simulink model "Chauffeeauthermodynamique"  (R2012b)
settings: Solver=ode45  StartTime=0.0  StopTime=60000  RelTol=1e-3
libraries: fl_lib x9, nesl_utility x6

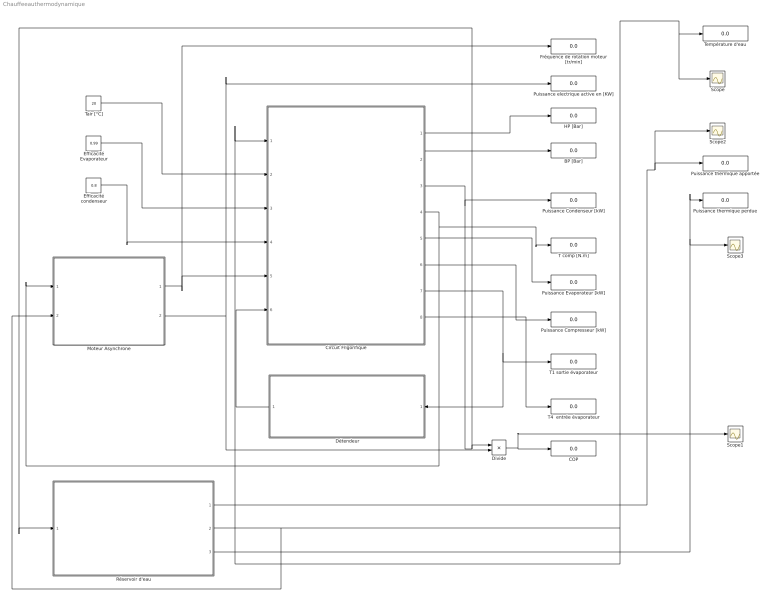
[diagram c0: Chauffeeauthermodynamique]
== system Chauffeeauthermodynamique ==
  BP [Bar] : Display
  COP : Display
  Circuit Frigorifique : Subsystem
  Divide : Product  Inputs=*/
  Détendeur : Subsystem
  Efficacité Evaporateur : Constant  Value=0.99
  Efficacité condenseur : Constant  Value=0.8
  Fréquence de rotation moteur [tr/min] : Display
  HP [Bar] : Display
  Moteur Asynchrone : Subsystem
  Puissance Compresseur [kW] : Display
  Puissance Condenseur [kW] : Display
  Puissance Evaporateur [kW] : Display
  Puissance electrique active en [KW] : Display
  Puissance thermique apportée : Display
  Puissance thermique perdue : Display
  Réservoir d'eau : Subsystem
  Scope{,1..3} (4 alike) : Scope
  T comp [N.m] : Display
  T1 sortie évaporateur : Display
  T4  entrée évaporateur : Display
  Tair [°C] : Constant  Value=20
  Température d'eau : Display
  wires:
  Efficacité Evaporateur/1 -> Circuit Frigorifique/3(Eff Evapo)
  Circuit Frigorifique/1(HP [bar]) -> HP [Bar]/1
  Circuit Frigorifique/2(BP [bar]) -> BP [Bar]/1
  Circuit Frigorifique/4(Tm [N.m]) -> Moteur Asynchrone/1(Tm [N.m]), T comp [N.m]/1
  Circuit Frigorifique/8(T4 [°C]) -> T4  entrée évaporateur/1
  Circuit Frigorifique/7(T1 [°C]) -> Détendeur/1(T1), T1 sortie évaporateur/1
  Circuit Frigorifique/5(Pevapo [kW]) -> Puissance Evaporateur [kW]/1
  Divide/1 -> Scope1/1, COP/1
  Circuit Frigorifique/6(Pcomp [kW]) -> Puissance Compresseur [kW]/1
  Efficacité condenseur/1 -> Circuit Frigorifique/4(effc)
  Détendeur/1(BP [Bar]) -> Circuit Frigorifique/6(BP[Bar])
  Moteur Asynchrone/2(Puissance Electrique active [W]) -> Puissance electrique active en [KW]/1, Divide/2
  Moteur Asynchrone/1(N [tr/min]) -> Fréquence de rotation moteur [tr/min]/1, Circuit Frigorifique/5(N [tr/min])
  Tair [°C]/1 -> Circuit Frigorifique/2(Tair [°C])
  Circuit Frigorifique/3(Pcond [kW]) -> Réservoir d'eau/1(" Puissance Condenseur [kW]"), Divide/1, Puissance Condenseur [kW]/1
  Réservoir d'eau/2(Température du réservoir [°C]) -> Moteur Asynchrone/2(Teau [°C]), Scope/1, Température d'eau/1, Circuit Frigorifique/1(Tee [°C])
  Réservoir d'eau/1(Puissance Condenseur [W]) -> Scope2/1, Puissance thermique apportée/1
  Réservoir d'eau/3(Puissance thermique perdue [W]) -> Scope3/1, Puissance thermique perdue/1

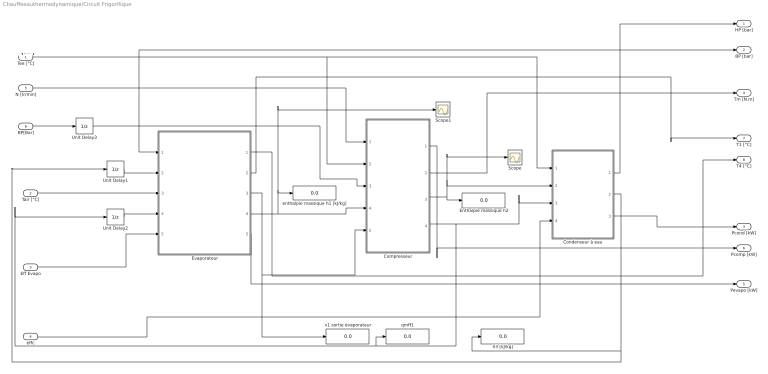
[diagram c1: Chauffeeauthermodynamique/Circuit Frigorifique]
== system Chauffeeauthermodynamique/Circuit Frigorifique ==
  note: +++++
  Tee [°C] : Inport
  Tair [°C] : Inport  Port=2
  Eff Evapo : Inport  Port=3
  effc : Inport  Port=4
  N [tr/min] : Inport  Port=5
  BP[Bar] : Inport  Port=6
  Compresseur : Subsystem
  Condenseur à eau : Subsystem
  Enthalpie massique h2 : Display
  Evaporateur : Subsystem
  Scope : Scope
  Scope1 : Scope
  Unit Delay1 : UnitDelay  InitialCondition=300  SampleTime=-1
  Unit Delay2 : UnitDelay  InitialCondition=0.00001  SampleTime=-1
  Unit Delay3 : UnitDelay  InitialCondition=2.5  SampleTime=-1
  enthalpie massique h1 [kJ/kg] : Display
  h3 [kJ/kg] : Display
  qmff1 : Display
  v1 sortie évaporateur : Display
  HP [bar] : Outport
  BP [bar] : Outport  Port=2
  Pcond [kW] : Outport  Port=3
  Tm [N.m] : Outport  Port=4
  Pevapo [kW] : Outport  Port=5
  Pcomp [kW] : Outport  Port=6
  T1 [°C] : Outport  Port=7
  T4 [°C] : Outport  Port=8
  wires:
  Evaporateur/2(T1 [°C]) -> T1 [°C]/1
  N [tr/min]/1 -> Compresseur/1(N [tr/min])
  Evaporateur/5(Pévapo [kW]) -> Pevapo [kW]/1
  Tair [°C]/1 -> Evaporateur/3(Tair [°C])
  Unit Delay2/1 -> Evaporateur/4(qmff [kg/s])
  Condenseur à eau/1(HP [bar]) -> HP [bar]/1
  BP[Bar]/1 -> Unit Delay3/1
  Compresseur/4(qmff [kg/s]) -> Unit Delay2/1, qmff1/1, Condenseur à eau/3(qmff [kg/s])
  Tee [°C]/1 -> Compresseur/2(Tee [°C]), Condenseur à eau/1(Tee [°C])
  Eff Evapo/1 -> Evaporateur/5(Eff)
  Evaporateur/3(v1 [m3/kg]) -> v1 sortie évaporateur/1, Compresseur/5(v1 [m3/kg])
  Condenseur à eau/2(h3 [kJ/kg]) -> Unit Delay1/1, h3 [kJ/kg]/1
  Evaporateur/4(h1 [kJ/kg]) -> Compresseur/4(h1 [kJ/kg]), Scope1/1, enthalpie massique h1 [kJ/kg]/1
  Compresseur/3(h2 [kJ/kg]) -> Scope/1, Condenseur à eau/2(h2 [kJ/kg]), Enthalpie massique h2/1
  Compresseur/2(Tm [N.m]) -> Tm [N.m]/1
  Evaporateur/1(T4 [°C]) -> T4 [°C]/1
  Condenseur à eau/3(Pcond [kW]) -> Pcond [kW]/1
  Unit Delay1/1 -> Evaporateur/2(h3 [kJ/kg])
  Compresseur/1(Pcomp [kW]) -> Pcomp [kW]/1
  effc/1 -> Condenseur à eau/4(effc)
  Unit Delay3/1 -> BP [bar]/1, Compresseur/3(BP [bar]), Evaporateur/1(BP [bar])

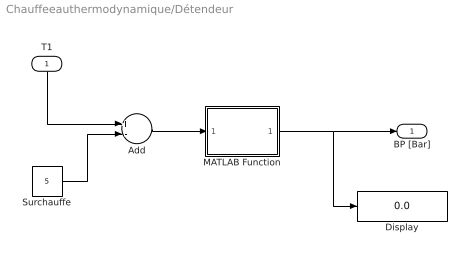
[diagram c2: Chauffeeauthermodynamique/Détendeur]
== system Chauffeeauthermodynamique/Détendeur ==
  T1 : Inport
  Add : Sum  Inputs=+-
  Display : Display
  MATLAB Function : MATLAB Function  TreatAsAtomicUnit=on
  Surchauffe : Constant  Value=5
  BP [Bar] : Outport
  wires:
  Add/1 -> MATLAB Function/1(T)
  T1/1 -> Add/1
  Surchauffe/1 -> Add/2
  MATLAB Function/1(BP) -> Display/1, BP [Bar]/1

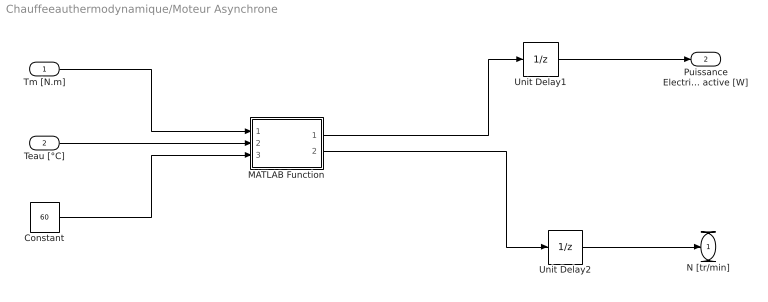
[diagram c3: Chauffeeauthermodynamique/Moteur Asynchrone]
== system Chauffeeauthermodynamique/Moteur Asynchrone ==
  Tm [N.m] : Inport
  Teau [°C] : Inport  Port=2
  Constant : Constant  Value=60
  MATLAB Function : MATLAB Function  TreatAsAtomicUnit=on
  Unit Delay1 : UnitDelay  InitialCondition=0.2  SampleTime=-1
  Unit Delay2 : UnitDelay  SampleTime=-1
  N [tr/min] : Outport
  Puissance Electrique active [W] : Outport  Port=2
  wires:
  Tm [N.m]/1 -> MATLAB Function/1(Tm)
  MATLAB Function/1(P) -> Unit Delay1/1
  MATLAB Function/2(N) -> Unit Delay2/1
  Unit Delay1/1 -> Puissance Electrique active [W]/1
  Unit Delay2/1 -> N [tr/min]/1
  Teau [°C]/1 -> MATLAB Function/2(Teau)
  Constant/1 -> MATLAB Function/3(Tcons)

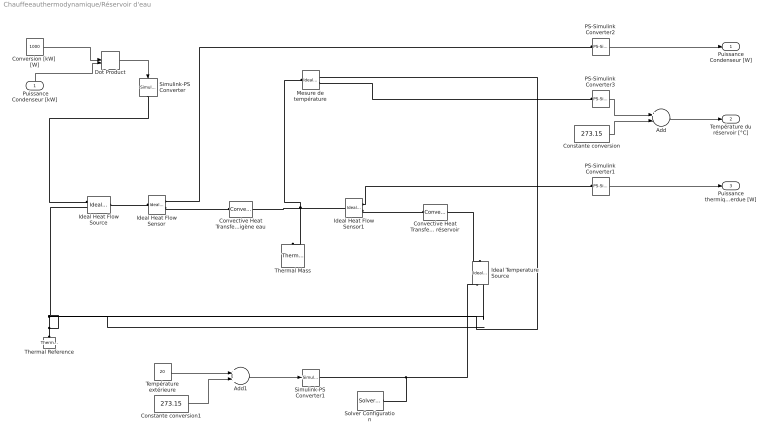
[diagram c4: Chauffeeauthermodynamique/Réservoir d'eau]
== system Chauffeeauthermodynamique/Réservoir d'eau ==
  " Puissance Condenseur [kW]" : Inport
  Add : Sum  Inputs=+-
  Add1 : Sum
  Constante conversion : Constant  Value=273.15
  Constante conversion1 : Constant  Value=273.15
  Convective Heat Transfer Echange Fluide frigorigène eau : fl_lib/Thermal/Thermal Elements/Convective Heat Transfer  area=0.82 m^2  heat_tr_coeff=25 W/(m^2 * K)  Q_Log=off  T_Log=off  LocalVarNames=|Q|T  LocalVarDescs=|Q|T  LocalVarLogging=[0 0]
  Convective Heat Transfer1 Echange avec l'extérieur du réservoir : fl_lib/Thermal/Thermal Elements/Convective Heat Transfer  area=1 m^2  heat_tr_coeff=0.0015 W/(m^2 * K)  Q_Log=off  T_Log=off  LocalVarNames=|Q|T  LocalVarDescs=|Q|T  LocalVarLogging=[0 0]
  Conversion [kW]  [W] : Constant  Value=1000
  Dot Product : DotProduct
  Ideal Heat Flow Sensor : fl_lib/Thermal/Thermal Sensors/Ideal Heat Flow Sensor  Q_Log=off  T_Log=off  LocalVarNames=|Q|T  LocalVarDescs=|Q|T  LocalVarLogging=[0 0]
  Ideal Heat Flow Sensor1 : fl_lib/Thermal/Thermal Sensors/Ideal Heat Flow Sensor  Q_Log=off  T_Log=off  LocalVarNames=|Q|T  LocalVarDescs=|Q|T  LocalVarLogging=[0 0]
  Ideal Heat Flow Source : fl_lib/Thermal/Thermal Sources/Ideal Heat Flow Source  Q_Log=off  T_Log=off  LocalVarNames=|Q|T  LocalVarDescs=|Q|T  LocalVarLogging=[0 0]
  Ideal Temperature Source : fl_lib/Thermal/Thermal Sources/Ideal Temperature Source  Q_Log=off  T_Log=off  LocalVarNames=|Q|T  LocalVarDescs=|Q|T  LocalVarLogging=[0 0]
  Mesure de température : fl_lib/Thermal/Thermal Sensors/Ideal Temperature Sensor  Qs_Log=off  Ts_Log=off  LocalVarNames=|Qs|Ts  LocalVarDescs=|Qs|Ts  LocalVarLogging=[]
  PS-Simulink Converter1 : nesl_utility/PS-Simulink Converter  PhysicalDomain=network_engine_domain  LeftPortType=input  RightPortType=output  SubClassName=ps_output  PseudoPeriodic=off  Frequencies=[]  Unit=1  AffineConversion=off
  PS-Simulink Converter2 : nesl_utility/PS-Simulink Converter  PhysicalDomain=network_engine_domain  LeftPortType=input  RightPortType=output  SubClassName=ps_output  PseudoPeriodic=off  Frequencies=[]  Unit=1  AffineConversion=off
  PS-Simulink Converter3 : nesl_utility/PS-Simulink Converter  PhysicalDomain=network_engine_domain  LeftPortType=input  RightPortType=output  SubClassName=ps_output  PseudoPeriodic=off  Frequencies=[]  Unit=1  AffineConversion=off
  Simulink-PS Converter : nesl_utility/Simulink-PS Converter  PhysicalDomain=network_engine_domain  LeftPortType=input  RightPortType=output  SubClassName=ps_input  PseudoPeriodic=off  Frequencies=[]  NoiseDistribution=none  NoiseParameters=[]  Unit=1  AffineConversion=off  InputFilterTimeConstant=.001  UdotUserProvided=1  SimscapeFilterOrder=1  InputFiltering=off
  Simulink-PS Converter1 : nesl_utility/Simulink-PS Converter  PhysicalDomain=network_engine_domain  LeftPortType=input  RightPortType=output  SubClassName=ps_input  PseudoPeriodic=off  Frequencies=[]  NoiseDistribution=none  NoiseParameters=[]  Unit=K  AffineConversion=on  InputFilterTimeConstant=.001  UdotUserProvided=1  SimscapeFilterOrder=1  InputFiltering=off
  Solver Configuration : nesl_utility/Solver Configuration  PhysicalDomain=network_engine_domain  LeftPortType=input  RightPortType=generic  SubClassName=solver  Accelerate=off  Profile=off  UseLocalSampling=off  FrequencyDomain=off  Tones=[]  Harmonics=[]  UseCCode=off  SimulateNoise=off  EnableSwitchedLinearOptims=on  DoDC=off  ResidualTolerance=1e-9  UseLocalSolver=off  LocalSolverChoice=NE_BACKWARD_EULER_ADVANCER  LocalSolverSampleTime=.001  DoFixedCost=off  MaxNonlinIter=3  MaxModeIter=2  LinearAlgebra=Sparse  DelaysMemoryBudget=1024
  Température extérieure : Constant  Value=20
  Thermal Mass : fl_lib/Thermal/Thermal Elements/Thermal Mass  mass=200 kg  sp_heat=4185 J/kg/K  init_temp=15 C  Q_Log=off  LocalVarNames=|Q  LocalVarDescs=|Q  LocalVarLogging=0
  Thermal Reference : fl_lib/Thermal/Thermal Elements/Thermal Reference  Q_Log=off  LocalVarNames=|Q  LocalVarDescs=|Q  LocalVarLogging=0
  Puissance Condenseur [W] : Outport
  Température du réservoir [°C] : Outport  Port=2
  Puissance thermique perdue [W] : Outport  Port=3
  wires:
  " Puissance Condenseur [kW]"/1 -> Dot Product/2
  PS-Simulink Converter3/1 -> Add/1
  Add/1 -> Température du réservoir [°C]/1
  Constante conversion/1 -> Add/2
  Dot Product/1 -> Simulink-PS Converter/1
  Conversion [kW]  [W]/1 -> Dot Product/1
  PS-Simulink Converter1/1 -> Puissance thermique perdue [W]/1
  PS-Simulink Converter2/1 -> Puissance Condenseur [W]/1
  Add1/1 -> Simulink-PS Converter1/1
  Température extérieure/1 -> Add1/1
  Constante conversion1/1 -> Add1/2
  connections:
  Thermal Reference/LConn1 -- Ideal Temperature Source/RConn2 -- Mesure de température/RConn1 -- Ideal Heat Flow Source/RConn2
  Mesure de température/LConn1 -- Thermal Mass/LConn1 -- Ideal Heat Flow Sensor1/LConn1 -- Convective Heat Transfer Echange Fluide frigorigène eau/RConn1
  Solver Configuration/RConn1 -- Ideal Temperature Source/RConn1 -- Simulink-PS Converter1/RConn1
  Simulink-PS Converter/RConn1 -- Ideal Heat Flow Source/RConn1
  Convective Heat Transfer1 Echange avec l'extérieur du réservoir/RConn1 -- Ideal Temperature Source/LConn1
  PS-Simulink Converter3/LConn1 -- Mesure de température/RConn2
  Ideal Heat Flow Source/LConn1 -- Ideal Heat Flow Sensor/LConn1
  Ideal Heat Flow Sensor/RConn2 -- Convective Heat Transfer Echange Fluide frigorigène eau/LConn1
  Ideal Heat Flow Sensor1/RConn2 -- Convective Heat Transfer1 Echange avec l'extérieur du réservoir/LConn1
  Ideal Heat Flow Sensor1/RConn1 -- PS-Simulink Converter1/LConn1
  Ideal Heat Flow Sensor/RConn1 -- PS-Simulink Converter2/LConn1

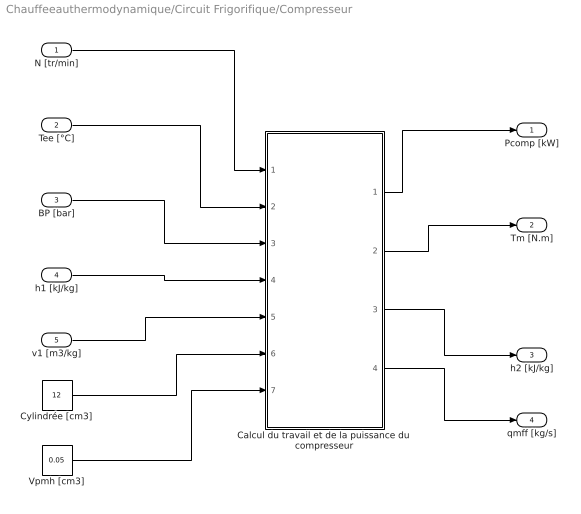
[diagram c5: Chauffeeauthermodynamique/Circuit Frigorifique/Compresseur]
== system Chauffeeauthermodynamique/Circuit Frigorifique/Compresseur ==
  N [tr/min] : Inport
  Tee [°C] : Inport  Port=2
  BP [bar] : Inport  Port=3
  h1 [kJ/kg] : Inport  Port=4
  v1 [m3/kg] : Inport  Port=5
  Calcul du travail et de la puissance du compresseur : MATLAB Function  TreatAsAtomicUnit=on
  Cylindrée [cm3] : Constant  Value=12
  Vpmh [cm3] : Constant  Value=0.05
  Pcomp [kW] : Outport
  Tm [N.m] : Outport  Port=2
  h2 [kJ/kg] : Outport  Port=3
  qmff [kg/s] : Outport  Port=4
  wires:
  Calcul du travail et de la puissance du compresseur/4(qmff) -> qmff [kg/s]/1
  Calcul du travail et de la puissance du compresseur/2(Tm) -> Tm [N.m]/1
  h1 [kJ/kg]/1 -> Calcul du travail et de la puissance du compresseur/4(h1)
  Tee [°C]/1 -> Calcul du travail et de la puissance du compresseur/2(Tee)
  BP [bar]/1 -> Calcul du travail et de la puissance du compresseur/3(BP)
  Calcul du travail et de la puissance du compresseur/1(P) -> Pcomp [kW]/1
  Calcul du travail et de la puissance du compresseur/3(h2) -> h2 [kJ/kg]/1
  N [tr/min]/1 -> Calcul du travail et de la puissance du compresseur/1(N)
  v1 [m3/kg]/1 -> Calcul du travail et de la puissance du compresseur/5(v1)
  Cylindrée [cm3]/1 -> Calcul du travail et de la puissance du compresseur/6(cyl)
  Vpmh [cm3]/1 -> Calcul du travail et de la puissance du compresseur/7(Vpmh)

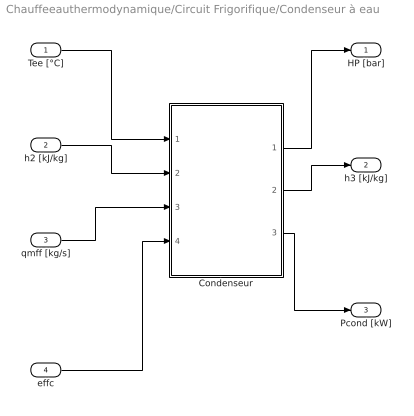
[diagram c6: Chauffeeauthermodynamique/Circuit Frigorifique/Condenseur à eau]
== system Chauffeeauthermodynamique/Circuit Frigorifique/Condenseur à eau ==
  Tee [°C] : Inport
  h2 [kJ/kg] : Inport  Port=2
  qmff [kg/s] : Inport  Port=3
  effc : Inport  Port=4
  Condenseur : MATLAB Function  TreatAsAtomicUnit=on
  HP [bar] : Outport
  h3 [kJ/kg] : Outport  Port=2
  Pcond [kW] : Outport  Port=3
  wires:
  Tee [°C]/1 -> Condenseur/1(Tee)
  Condenseur/1(HP) -> HP [bar]/1
  h2 [kJ/kg]/1 -> Condenseur/2(h2)
  qmff [kg/s]/1 -> Condenseur/3(qmff)
  Condenseur/2(h3) -> h3 [kJ/kg]/1
  Condenseur/3(Pcond) -> Pcond [kW]/1
  effc/1 -> Condenseur/4(eff)

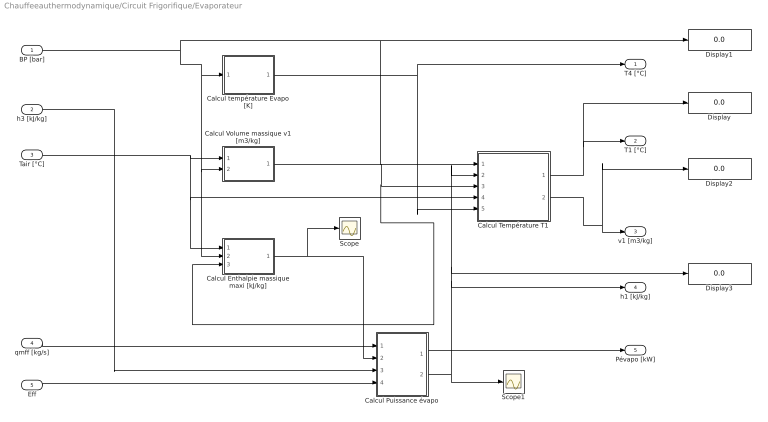
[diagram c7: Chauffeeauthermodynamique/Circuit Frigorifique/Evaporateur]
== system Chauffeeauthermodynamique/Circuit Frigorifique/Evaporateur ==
  BP [bar] : Inport
  h3 [kJ/kg] : Inport  Port=2
  Tair [°C] : Inport  Port=3
  qmff [kg/s] : Inport  Port=4
  Eff : Inport  Port=5
  Calcul Enthalpie massique maxi [kJ/kg] : MATLAB Function  TreatAsAtomicUnit=on
  Calcul Puissance évapo : MATLAB Function  TreatAsAtomicUnit=on
  Calcul Température T1 : MATLAB Function  TreatAsAtomicUnit=on
  Calcul Volume massique v1 [m3/kg] : MATLAB Function  TreatAsAtomicUnit=on
  Calcul température Evapo [K] : MATLAB Function  TreatAsAtomicUnit=on
  Display{,1..3} (4 alike) : Display
  Scope : Scope
  Scope1 : Scope
  T4 [°C] : Outport
  T1 [°C] : Outport  Port=2
  v1 [m3/kg] : Outport  Port=3
  h1 [kJ/kg] : Outport  Port=4
  Pévapo [kW] : Outport  Port=5
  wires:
  qmff [kg/s]/1 -> Calcul Puissance évapo/1(qmff)
  Calcul Enthalpie massique maxi [kJ/kg]/1(H) -> Scope/1, Calcul Puissance évapo/2(hmax)
  BP [bar]/1 -> Calcul Enthalpie massique maxi [kJ/kg]/2(P), Calcul Volume massique v1 [m3/kg]/2(P), Calcul température Evapo [K]/1(P), Display1/1, Calcul Température T1/1(P)
  Calcul température Evapo [K]/1(T) -> T4 [°C]/1, Calcul Température T1/5(T3)
  Tair [°C]/1 -> Calcul Enthalpie massique maxi [kJ/kg]/1(T), Calcul Température T1/4(T1max), Calcul Volume massique v1 [m3/kg]/1(T)
  Calcul Puissance évapo/1(Pevapo) -> Pévapo [kW]/1
  Eff/1 -> Calcul Puissance évapo/4(eff)
  Calcul Volume massique v1 [m3/kg]/1(v) -> Calcul Enthalpie massique maxi [kJ/kg]/3(v), Calcul Température T1/3(v)
  Calcul Température T1/2(v1) -> Display2/1, v1 [m3/kg]/1
  Calcul Température T1/1(T1) -> Display/1, T1 [°C]/1
  Calcul Puissance évapo/2(h1) -> h1 [kJ/kg]/1, Display3/1, Calcul Température T1/2(h), Scope1/1
  h3 [kJ/kg]/1 -> Calcul Puissance évapo/3(h3)
